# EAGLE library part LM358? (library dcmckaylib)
Cheap dual op-amp
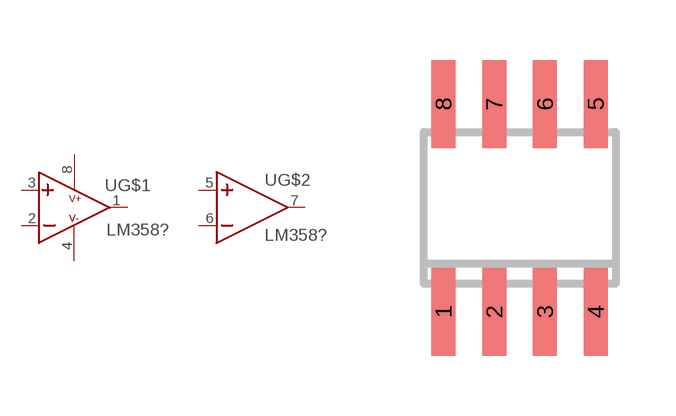
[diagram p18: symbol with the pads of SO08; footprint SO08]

Designator prefix -; gates G$1=OPAMP2 G$2=OPAMP

## LM358  [SO08]
1  G$1:OUT  out
2  G$1:IN-  in
3  G$1:IN+  in
4  G$1:V-  pwr
5  G$2:IN+  in
6  G$2:IN-  in
7  G$2:OUT  out
8  G$1:V+  pwr

## Footprint SO08 (pad centres in mm)
Small Outline Package 8 NS Package M08A
smd 0.6 x 2.2: 1 -1.905,-2.6; 2 -0.635,-2.6; 3 0.635,-2.6; 4 1.905,-2.6; 5 1.905,2.6; 6 0.635,2.6; 7 -0.635,2.6; 8 -1.905,2.6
